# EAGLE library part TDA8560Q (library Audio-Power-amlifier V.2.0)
2x40W Stereo BTL Amplifier
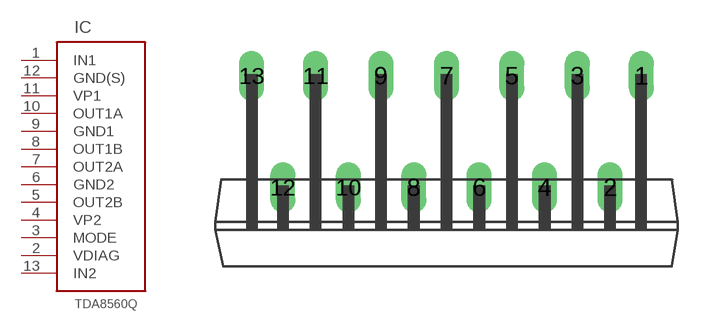
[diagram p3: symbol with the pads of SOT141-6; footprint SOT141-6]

Designator prefix IC

## TDA8560Q  [SOT141-6]
1  IN1
2  VDIAG
3  MODE
4  VP2
5  OUT2B
6  GND2
7  OUT2A
8  OUT1B
9  GND1
10  OUT1A
11  VP1
12  GND(S)
13  IN2

## Footprint SOT141-6 (pad centres in mm)
drill 0.8 long: 1 10.12,5.8; 2 8.5,0; 3 6.8,5.8; 4 5.1,0; 5 3.4,5.8; 6 1.7,0; 7 0,5.8; 8 -1.7,0; 9 -3.4,5.8; 10 -5.1,0; 11 -6.8,5.8; 12 -8.5,0; 13 -10.12,5.8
